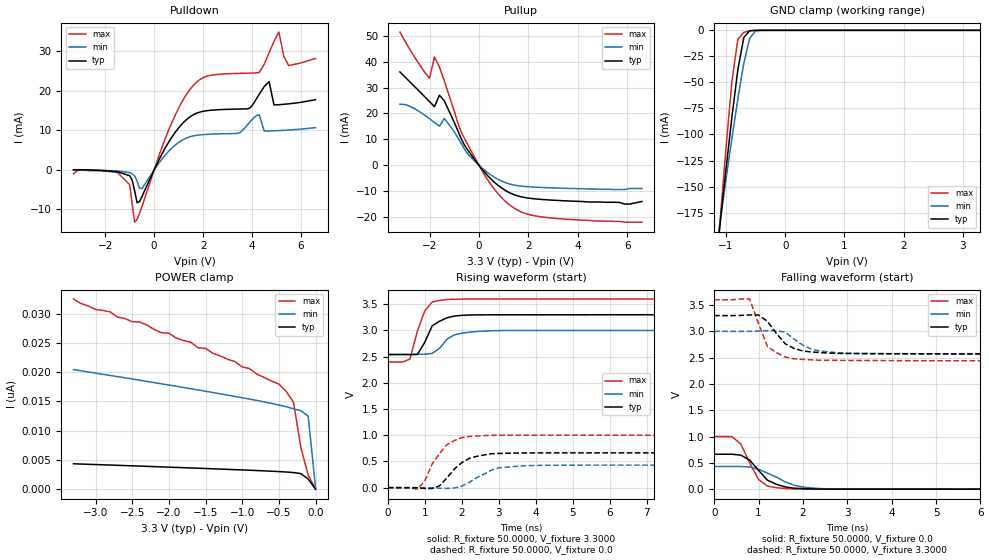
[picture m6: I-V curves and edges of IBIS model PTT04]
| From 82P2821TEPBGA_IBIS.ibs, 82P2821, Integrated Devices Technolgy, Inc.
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|   Model PTT04
[Model]		PTT04
Model_type	3-state
Polarity   Non-Inverting
Enable   Active-Low
C_comp   5.4700pF   4.8200pF   6.1000pF
[Temperature Range]	  25.0000   90.0000   -40.0000
[Voltage Range]   3.3000V   3.0000V   3.6000V
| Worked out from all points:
|   slope of the pulldown table from 0 to 0.495 V, typ, clamps not added: 82.7 ohm
|   slope of the pullup table from 0 to 0.495 V, typ, clamps not added: 91.5 ohm
|   GND clamp passes 1 mA (typ) near -0.61 V on its own axis
|   rising waveform, R_fixture 50.0000, V_fixture 3.3000: 20-80 % time 408ps typ, 428ps min, 324ps max; typ from 2.54 V to 3.3 V
|   rising waveform, R_fixture 50.0000, V_fixture 0.0: 20-80 % time 605ps typ, 685ps min, 530ps max; typ from 0 V to 0.664 V
|   falling waveform, R_fixture 50.0000, V_fixture 0.0: 20-80 % time 477ps typ, 672ps min, 357ps max; typ from 0.664 V to 0 V
|   falling waveform, R_fixture 50.0000, V_fixture 3.3000: 20-80 % time 481ps typ, 519ps min, 369ps max; typ from 3.3 V to 2.57 V
[Pulldown]
|Voltage	  I(typ)   I(min)   I(max)
-3.3V     0A         0A         -1mA
-1.5V     -500uA     -300uA     -700uA
-1V       -1.5mA     -700uA     -3.8mA
-800mV    -5.28mA    -1.58mA    -13.28mA
-500mV    -6.771mA   -4.745mA   -9.284mA
700mV     8.065mA    5.38mA     11.66mA
1.7V      14.26mA    8.709mA    22.03mA
4.3V      19.2mA     13.9mA     24.71mA
4.7V      22.37mA    9.863mA    29.69mA
5.1V      16.51mA    9.953mA    34.92mA
5.5V      16.73mA    10.09mA    26.45mA
6.6V      17.78mA    10.7mA     28.24mA
[Pullup]
|Voltage	  I(typ)   I(min)   I(max)
-3.2V     36.03mA    23.51mA    51.42mA
-2V       24.54mA    17.97mA    33.63mA
-1.8V     22.64mA    16.51mA    41.83mA
-1.6V     27.05mA    15.1mA     37.9mA
-1.4V     24.85mA    18.06mA    32.59mA
-700mV    9.882mA    8.072mA    12.47mA
-400mV    5.196mA    3.842mA    7.041mA
400mV     -4.493mA   -3.199mA   -6.275mA
1.2V      -10.42mA   -7.106mA   -15.02mA
1.8V      -12.37mA   -8.151mA   -18.37mA
2.6V      -13.26mA   -8.62mA    -20.02mA
6.6V      -14mA      -9mA       -22mA
[GND_clamp]
|Voltage	  I(typ)   I(min)   I(max)
-3.3V     -1.417A    -1.129A    -1.858A
-1.2V     -239.1mA   -224.9mA   -255mA
-1.1V     -185.6mA   -183.6mA   -182.5mA
-1V       -133.2mA   -143mA     -112.6mA
-900mV    -82.99mA   -103.4mA   -48.97mA
-800mV    -37.69mA   -65.64mA   -8.51mA
-700mV    -7.022mA   -31.73mA   -1.941mA
-600mV    -418.4uA   -7.67mA    -417.7uA
-500mV    -26.63uA   -550.4uA   -45.84uA
3.3V      790.7fA    13.73nA    -711.9pA
[POWER_clamp]
|Voltage	  I(typ)   I(min)   I(max)
-3.3V     4.337nA    20.42nA    32.48nA
-3V       4.207nA    19.83nA    30.71nA
-2.4V     3.943nA    18.62nA    28.56nA
-2.1V     3.806nA    18nA       26.73nA
-1.7V     3.623nA    17.16nA    25.11nA
-1.6V     3.577nA    16.95nA    24.14nA
-1.5V     3.53nA     16.73nA    24.06nA
-500mV    3.006nA    14.38nA    17.96nA
-300mV    2.841nA    13.73nA    14.83nA
-200mV    2.657nA    13.4nA     7.087nA
-100mV    1.727nA    12.47nA    2.401nA
0V        821.5fA    199.7pA    548fA
[Ramp]
| variable   typ   min   max
dV/dt_r		0.3985/0.5758n   0.2582/0.7146n   0.6000/0.4525n
dV/dt_f		0.4392/0.4283n   0.2598/0.4991n   0.6984/0.3242n
R_load =	50.0000
[Rising Waveform]
R_fixture=	50.0000
V_fixture=	3.3000
V_fixture_min=	3.0000
V_fixture_max=	3.6000
|time   V(typ)   V(min)   V(max)
0s        2.539V     2.545V     2.398V
600ps     2.539V     2.545V     2.455V
800ps     2.543V     2.545V     2.988V
1ns       2.774V     2.547V     3.372V
1.2ns     3.089V     2.562V     3.544V
1.4ns     3.175V     2.658V     3.574V
1.6ns     3.242V     2.833V     3.591V
1.8ns     3.275V     2.917V     3.596V
2.6ns     3.298V     2.988V     3.599V
10ns      3.3V       3V         3.599V
[Rising Waveform]
R_fixture=	50.0000
V_fixture=	0.0
V_fixture_min=	0.0
V_fixture_max=	0.0
|time   V(typ)   V(min)   V(max)
0s        0V         0V         0V
800ps     -2.276mV   75.54uV    -28.46mV
1ns       -14.88mV   -665.2uV   128.5mV
1.2ns     -15.4mV    -3.918mV   452.1mV
1.4ns     36.06mV    -10.13mV   650.2mV
1.6ns     187.6mV    -14.77mV   822.1mV
2.2ns     558.5mV    101.3mV    976.1mV
2.8ns     647.4mV    335mV      999.1mV
3.6ns     661.9mV    413.6mV    1V
10ns      664.1mV    430.3mV    1V
[Falling Waveform]
R_fixture=	50.0000
V_fixture=	0.0
V_fixture_min=	0.0
V_fixture_max=	0.0
|time   V(typ)   V(min)   V(max)
0s        664.1mV    430.4mV    1V
400ps     665.1mV    430.6mV    999.6mV
600ps     646.3mV    430.4mV    857.9mV
800ps     552.2mV    422mV      499mV
1ns       357.3mV    379mV      183.2mV
1.2ns     170.6mV    305.2mV    58.7mV
1.4ns     93.5mV     230.2mV    28.23mV
1.8ns     18.4mV     75.53mV    5.072mV
2.4ns     1.636mV    11.42mV    -22.75uV
10ns      -6.392uV   -4.88uV    -3.538uV
[Falling Waveform]
R_fixture=	50.0000
V_fixture=	3.3000
V_fixture_min=	3.0000
V_fixture_max=	3.6000
|time   V(typ)   V(min)   V(max)
0s        3.3V       3V         3.6V
800ps     3.312V     3.001V     3.614V
1ns       3.312V     3.006V     3.144V
1.2ns     3.189V     3.013V     2.711V
1.6ns     2.764V     2.986V     2.511V
1.8ns     2.676V     2.853V     2.479V
2ns       2.626V     2.736V     2.467V
2.2ns     2.607V     2.658V     2.458V
2.8ns     2.581V     2.59V      2.448V
10ns      2.568V     2.567V     2.436V
